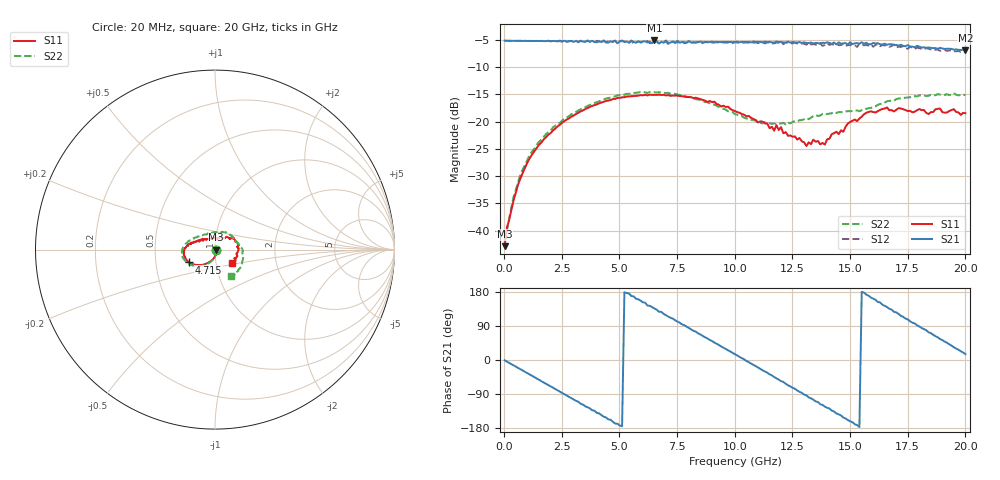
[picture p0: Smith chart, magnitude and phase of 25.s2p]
!Agilent Technologies,N5230A,US43500223,A.07.50.48
!Agilent N5230A: A.07.50.48
!Date: Thursday, October 08, 2015 12:15:02
!Correction: S11(Full 2 Port(1,2))
!S21(Full 2 Port(1,2))
!S12(Full 2 Port(1,2))
!S22(Full 2 Port(1,2))
!S2P File: Measurements: S11, S21, S12, S22:
# Hz S  dB  R 50
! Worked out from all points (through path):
!   201 points, 20 MHz to 20 GHz, reference 50 ohm
!   highest |S21| = -5.14 dB at 6.513 GHz (marker M1); lowest = -6.9 dB at 20 GHz (marker M2)
!   group delay of S21, straight-line fit = 97.5 ps
!   lowest |S11| = -42.9 dB at 20 MHz (marker M3), VSWR 1.01, Z = 50.7 - j0.0202 ohm
!   |S11| at or under -10 dB: start of sweep to end of sweep
!   |S22| runs from -42.1 to -14.6 dB; largest |S21 - S12| = 0.057
!   S11 on the Smith chart (normalised r, x): 20 MHz: 1.01, -0.00; 4.715 GHz: 0.74, -0.11; 20 GHz: 1.19, -0.18
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2e7  -42.85 -1.6  -5.18 -0.7  -5.19 -0.8  -42.07 -4.1
4.196e8  -34.26 -66.6  -5.22 -14.7  -5.22 -14.7  -33.66 -68.3
1.1189e9  -26.67 -96.6  -5.23 -38.7  -5.23 -38.9  -26.03 -96.8
2.3177e9  -20.89 -121.3  -5.27 -80.4  -5.29 -80.9  -20.53 -119.0
3.4166e9  -17.98 -137.2  -5.35 -117.5  -5.51 -119.0  -17.56 -135.4
4.7153e9  -15.89 -153.4  -5.43 -163.3  -5.32 -163.4  -15.50 -153.2
5.5145e9  -15.37 -162.4  -5.23 168.9  -5.15 168.4  -14.83 -163.0
6.5135e9  -15.10 -171.3  -5.14 136.3  -5.31 135.8  -14.64 -174.2
6.7133e9  -15.08 -172.1  -5.71 127.3  -5.64 126.1  -14.62 -175.8
8.012e9  -15.53 177.9  -5.25 84.5  -5.41 83.1  -15.53 169.8
1.001e10  -18.09 161.8  -5.42 15.1  -5.48 13.3  -18.64 141.3
1.08092e10  -19.54 151.6  -5.32 -12.8  -5.53 -14.4  -19.73 125.7
1.2008e10  -21.03 138.0  -5.41 -55.8  -5.45 -57.3  -20.36 96.6
1.31069e10  -24.50 106.3  -5.61 -93.3  -5.92 -96.2  -19.35 66.8
1.34066e10  -23.33 97.4  -5.69 -104.8  -5.81 -108.2  -19.03 59.8
1.39061e10  -24.23 79.2  -5.64 -123.1  -5.97 -124.9  -18.63 46.8
1.5005e10  -20.10 43.0  -5.46 -161.9  -6.03 -161.7  -18.12 26.7
1.59041e10  -18.12 24.3  -5.83 164.7  -5.86 163.4  -17.53 15.0
1.67033e10  -17.93 8.8  -5.83 135.1  -6.33 133.9  -16.20 -2.6
1.73027e10  -17.75 -2.2  -6.15 114.0  -6.19 110.4  -15.68 -17.3
1.83017e10  -18.41 -22.5  -6.47 78.6  -6.56 74.7  -15.35 -39.5
2e10  -18.48 -37.8  -6.93 15.7  -7.16 12.9  -15.19 -58.5
